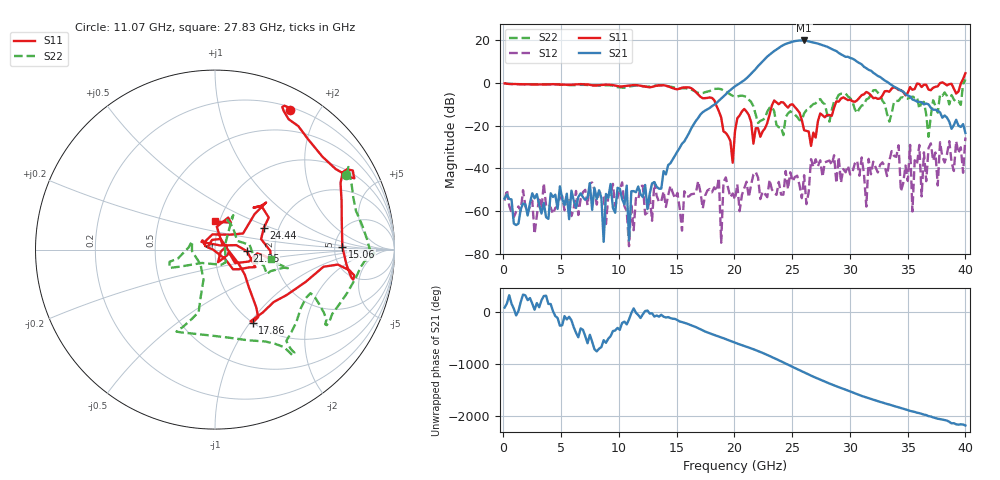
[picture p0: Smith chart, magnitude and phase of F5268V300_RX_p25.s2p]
!S2P File: Measurements: S11,S21,S12,S22
# MHz S  RI  R 50
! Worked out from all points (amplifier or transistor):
!   201 points, 100 MHz to 40 GHz, reference 50 ohm
!   highest |S21| = 19.9 dB at 26.04 GHz (marker M1)
!   |S21| within 3 dB of that: 23.98 GHz to 28.05 GHz (4.075 GHz wide, 15.7 % of centre)
!   unconditionally stable (mu >= 1): start of sweep to 37.83 GHz; 38.17 GHz to 39.69 GHz
!   at 6.684 GHz: K = 2198.27, MAG = -35.1 dB, |S12| = -54.4 dB
!   at 20.05 GHz: K = 246.75, MAG = -0.4 dB, |S12| = -54.6 dB
!   at 40 GHz: K = 121.54, MSG = 1.1 dB, |S12| = -25.6 dB
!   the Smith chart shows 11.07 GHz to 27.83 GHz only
!   S11 on the Smith chart (normalised r, x): 11.07 GHz: 0.24, +1.65; 15.06 GHz: 5.86, +0.37; 17.86 GHz: 1.00, -1.03; 21.25 GHz: 1.43, -0.02; 24.44 GHz: 1.67, +0.45; 27.83 GHz: 0.96, +0.31
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100  -0.9744 0.0448  2.48e-05 0.00195  -0.00171 -0.000343  -0.9856 0.0403
6883  -0.5579 0.7452  0.00196 0.000742  0.00148 0.00231  -0.1039 0.8944
11073  0.4175 0.7757  0.00278 -0.000823  -0.000513 -0.00138  0.732 0.4175
13467  0.7763 0.3974  0.000234 -0.00331  0.000833 -0.00139  0.8772 -0.0284
15063  0.7095 0.0158  -0.022 -0.0113  0.00262 -0.000327  0.696 -0.3002
17856  0.2099 -0.4064  0.1748 -0.1908  -0.00216 0.00244  0.3972 -0.5094
20050  0.055 -0.0504  -0.5418 0.6336  0.00144 -0.00118  -0.014 -0.4797
21247  0.1766 -0.00821  1.175 0.8519  0.00173 0.00117  -0.1274 -0.3849
22245  -0.0516 0.0177  1.855 -2.133  -0.00166 0.000914  -0.1286 -0.00728
23043  0.1564 0.0901  -2.78 -3.66  -0.00512 0.00154  -0.2534 -0.0679
23841  0.2143 0.2338  -5.81 3.227  -0.00174 0.00446  0.035 -0.0844
24439  0.2724 0.1225  0.5172 8.188  -0.00838 0.00195  0.0847 0.135
25237  0.2718 -0.0337  9.597 0.0681  0.00533 -0.00329  0.0681 0.1665
26035  0.0766 -0.0145  0.7959 -9.893  0.00617 -0.00302  0.1922 0.0273
26833  0.0657 0.0196  -8.704 -1.944  -0.0107 0.00083  0.2889 -0.1357
27432  0.0735 0.1783  -5.659 5.687  0.00573 0.0143  0.4059 -0.1036
27831  0.00182 0.157  -0.8923 7.287  -0.00798 0.0113  0.3104 -0.0502
28828  0.2347 0.2858  5.551 0.6816  0.00259 -0.00367  0.1333 -0.3937
29826  0.182 0.352  0.9937 -3.989  -0.00995 -0.00568  0.4116 -0.2529
30823  0.3955 0.2189  -2.807 -0.8072  0.00656 -0.00132  0.00938 -0.2502
33417  0.6195 0.0722  0.9509 0.2179  -0.00405 0.0147  -0.0508 0.1124
40000  1.433 -0.9017  0.0572 -0.0354  -0.00854 -0.0519  0.2341 -1.189
